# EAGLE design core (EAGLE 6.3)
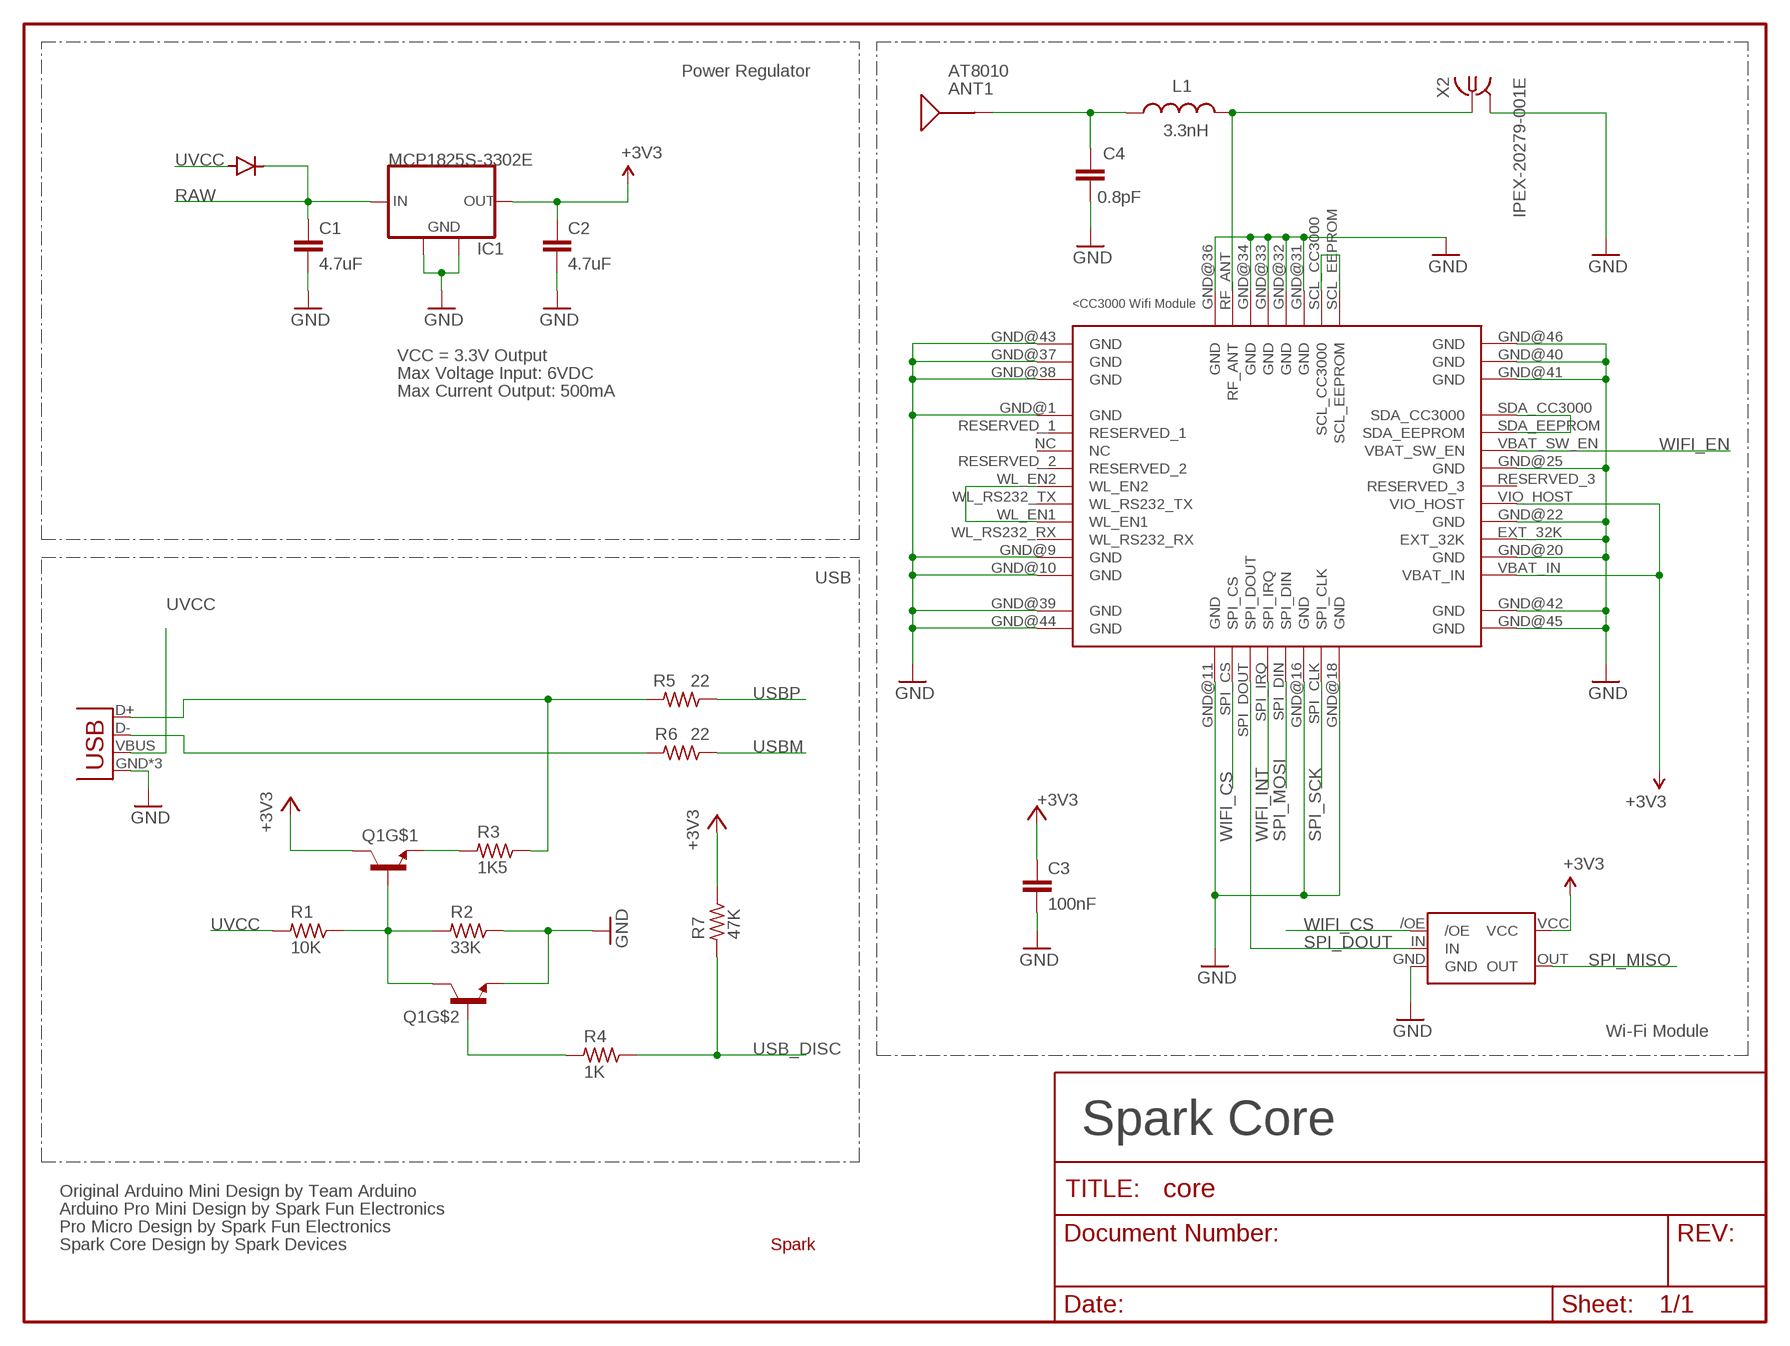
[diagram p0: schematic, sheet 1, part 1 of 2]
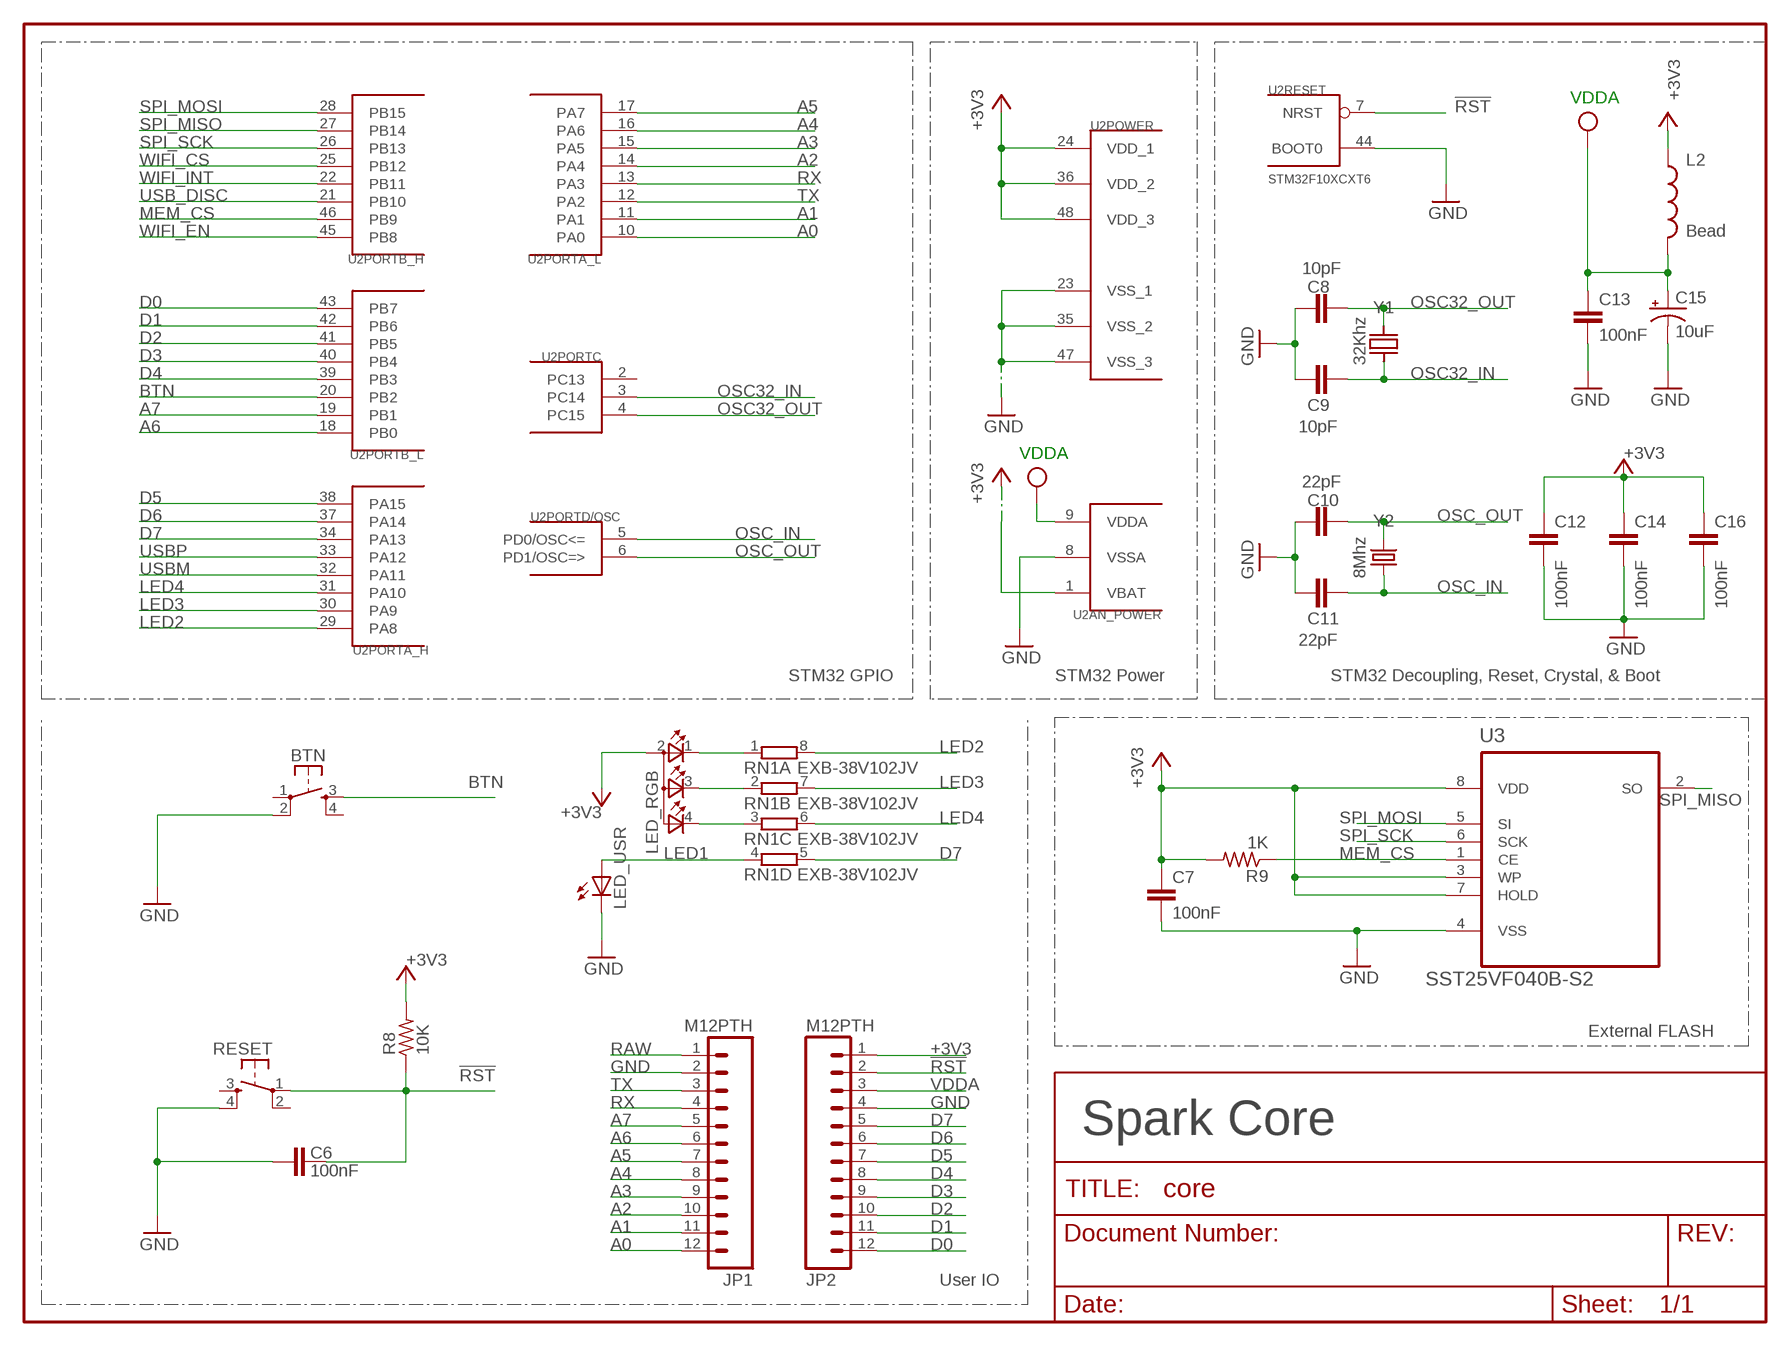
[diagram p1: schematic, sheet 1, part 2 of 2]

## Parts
ANT1  AT8010  [AT8010]
BTN  KMR211GLFS  TAC_SWITCHSMD  [TACTILE_SWITCH_SMD]
C1  4.7uF  C-EUC0603  [C0603]
C2  4.7uF  C-EUC0603  [C0603]
C3  100nF  C-EUC0603  [C0603]
C4  0.8pF  C-EUC0603  [C0603]
C6  100nF  C-EUC0603  [C0603]
C7  100nF  C-EUC0603  [C0603]
C8  10pF  C-EUC0603  [C0603]
C9  10pF  C-EUC0603  [C0603]
C10  22pF  C-EUC0603  [C0603]
C11  22pF  C-EUC0603  [C0603]
C12  100nF  C-EUC0603  [C0603]
C13  100nF  C-EUC0603  [C0603]
C14  100nF  C-EUC0603  [C0603]
C15  10uF  TANT-CAP1206  [EIA3216]
C16  100nF  C-EUC0603  [C0603]
D1  DIODE  [DIODE-DO-220AA(SMP)]
IC1  MCP1825S-3302E  MCP1825S-SOT223  [SOT223]
JP1  M12PTH  [1X12-SMALL-PADS]
JP2  M12PTH  [1X12-SMALL-PADS]
L1  3.3nH  INDUCTOR0603  [0603]
L2  Bead  INDUCTOR0603  [0603]
LED_RGB  TOPLED-3PLCC  [P-LCC-4-3]
LED_USR  LED0603  [LED-0603]
Q1  MMDT3904  [SOT363]
R1  10K  R-US_R0603  [R0603]
R2  33K  R-US_R0603  [R0603]
R3  1K5  R-US_R0603  [R0603]
R4  1K  R-US_R0603  [R0603]
R5  22  R-US_R0603  [R0603]
R6  22  R-US_R0603  [R0603]
R7  47K  R-US_R0603  [R0603]
R8  10K  R-US_R0603  [R0603]
R9  1K  R-US_R0603  [R0603]
RESET  KMR211GLFS  TAC_SWITCHSMD  [TACTILE_SWITCH_SMD]
RN1  EXB-38V102JV  4R-NEXB38V  [EXB38V]
U1  CC3000  [CC3000]
U2  STM32F10XCXT6  [TQFP48]
U3  SST25VF040B-S2  [SOIC127P790X216-8N]
U4  NL17SZ125SOT553  [SOT-553]
U$1  SPARK_LOGO2  [SPARK_LOGO2]
X1  USB-MICROB  USBUSB-MICROB-SLOT-HOLE  [USB-MICROB-SLOT-HOLE]
X2  IPEX-20279-001E  [IPEX-20279-001E]
Y1  32Khz  Q_FC135  [FC135]
Y2  8Mhz  CRYSTAL5X3  [CRYSTAL-SMD-5X3]

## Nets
!RST: C6.2 JP2.2 R8.1 RESET.1 U2.7(RESET:NRST)
+3V3: C2.1 C3.1 C7.1 C12.1 C14.1 C16.1 IC1.3(OUT) JP2.1 L2.1 LED_RGB.2(A2) Q1.3(C) R7.1 R8.2 R9.2 U1.VBAT_IN U1.VIO_HOST U2.1(AN_POWER:VBAT) U2.24(POWER:VDD_1) U2.36(POWER:VDD_2) U2.48(POWER:VDD_3) U3.3(WP) U3.7(HOLD) U3.8(VDD) U4.VCC
A0: JP1.12 U2.10(PORTA_L:PA0)
A1: JP1.11 U2.11(PORTA_L:PA1)
A2: JP1.10 U2.14(PORTA_L:PA4)
A3: JP1.9 U2.15(PORTA_L:PA5)
A4: JP1.8 U2.16(PORTA_L:PA6)
A5: JP1.7 U2.17(PORTA_L:PA7)
A6: JP1.6 U2.18(PORTB_L:PB0)
A7: JP1.5 U2.19(PORTB_L:PB1)
BTN: BTN.3 U2.20(PORTB_L:PB2)
D0: JP2.12 U2.43(PORTB_L:PB7)
D1: JP2.11 U2.42(PORTB_L:PB6)
D2: JP2.10 U2.41(PORTB_L:PB5)
D3: JP2.9 U2.40(PORTB_L:PB4)
D4: JP2.8 U2.39(PORTB_L:PB3)
D5: JP2.7 U2.38(PORTA_H:PA15)
D6: JP2.6 U2.37(PORTA_H:PA14)
D7: JP2.5 RN1.5 U2.34(PORTA_H:PA13)
GND [vcc]: BTN.2 C1.2 C2.2 C3.2 C4.2 C6.1 C7.2 C8.2 C9.2 C10.2 C11.2 C12.2 C13.2 C14.2 C15.C(-) C16.2 IC1.2(GND) IC1.4(GND) JP1.2 JP2.4 LED_USR.C Q1.1(E) R2.1 RESET.4 U1.EXT_32K U1.GND@1(GND) U1.GND@9(GND) U1.GND@10(GND) U1.GND@11(GND) U1.GND@16(GND) U1.GND@18(GND) U1.GND@20(GND) U1.GND@22(GND) U1.GND@25(GND) U1.GND@31(GND) U1.GND@32(GND) U1.GND@33(GND) U1.GND@34(GND) U1.GND@36(GND) U1.GND@37(GND) U1.GND@38(GND) U1.GND@39(GND) U1.GND@40(GND) U1.GND@41(GND) U1.GND@42(GND) U1.GND@43(GND) U1.GND@44(GND) U1.GND@45(GND) U1.GND@46(GND) U2.8(AN_POWER:VSSA) U2.23(POWER:VSS_1) U2.35(POWER:VSS_2) U2.44(RESET:BOOT0) U2.47(POWER:VSS_3) U3.4(VSS) U4.GND X1.GND X1.MT1(GND) X1.MT2(GND) X2.2@1(GND) X2.2@2(GND)
LED1: LED_USR.A RN1.4
LED2: RN1.8 U2.29(PORTA_H:PA8)
LED3: RN1.7 U2.30(PORTA_H:PA9)
LED4: RN1.6 U2.31(PORTA_H:PA10)
MEM_CS: R9.1 U2.46(PORTB_H:PB9) U3.1(CE)
N$1: R3.1 R5.2 X1.D+
N$2 [RF]: L1.2 U1.RF_ANT X2.1
N$3 [RF]: ANT1.SIG(SIGNAL) C4.1 L1.1
N$6: R6.2 X1.D-
N$7: U1.SCL_CC3000 U1.SCL_EEPROM
N$8: Q1.2(B) R4.2
N$9: U1.WL_EN1 U1.WL_EN2
N$10: LED_RGB.1(CRED) RN1.1
N$12: LED_RGB.3(CBLUE) RN1.2
N$13: Q1.5(B) Q1.6(C) R1.1 R2.2
N$14: LED_RGB.4(CGREEN) RN1.3
N$15: U1.SDA_CC3000 U1.SDA_EEPROM
N$16: Q1.4(E) R3.2
OSC32_IN: C9.1 U2.3(PORTC:PC14) Y1.X1
OSC32_OUT: C8.1 U2.4(PORTC:PC15) Y1.X2
OSC_IN: C11.1 U2.5(PORTD/OSC:PD0/OSC<=) Y2.1
OSC_OUT: C10.1 U2.6(PORTD/OSC:PD1/OSC=>) Y2.3
RAW [vcc]: C1.1 D1.CATHODE IC1.1(IN) JP1.1
RX: JP1.4 U2.13(PORTA_L:PA3)
SPI_DOUT: U1.SPI_DOUT U4.IN
SPI_MISO: U2.27(PORTB_H:PB14) U3.2(SO) U4.OUT
SPI_MOSI: U1.SPI_DIN U2.28(PORTB_H:PB15) U3.5(SI)
SPI_SCK: U1.SPI_CLK U2.26(PORTB_H:PB13) U3.6(SCK)
TX: JP1.3 U2.12(PORTA_L:PA2)
USB_DISC: R4.1 R7.2 U2.21(PORTB_H:PB10)
USBM: R6.1 U2.32(PORTA_H:PA11)
USBP: R5.1 U2.33(PORTA_H:PA12)
UVCC: D1.ANODE R1.2 X1.VBUS
VDDA: C13.1 C15.A(+) JP2.3 L2.2 U2.9(AN_POWER:VDDA) ; supply symbol labelled VCC
WIFI_CS: U1.SPI_CS U2.25(PORTB_H:PB12) U4./OE
WIFI_EN: U1.VBAT_SW_EN U2.45(PORTB_H:PB8)
WIFI_INT: U1.SPI_IRQ U2.22(PORTB_H:PB11)
Unconnected: BTN.1 BTN.4 RESET.2 RESET.3 U1.NC U1.RESERVED_1 U1.RESERVED_2 U1.RESERVED_3 U1.WL_RS232_RX U1.WL_RS232_TX U2.2(PORTC:PC13)

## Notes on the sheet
- Power Regulator
- VDDA
- VCC = 3.3V Output
- Max Voltage Input: 6VDC
- Max Current Output: 500mA
- VDDA
- USB
- STM32 GPIO | STM32 Power | STM32 Decoupling, Reset, Crystal, & Boot
- Wi-Fi Module | External FLASH
- Spark Core | Spark Core
- Original Arduino Mini Design by Team Arduino
- Arduino Pro Mini Design by Spark Fun Electronics
- Pro Micro Design by Spark Fun Electronics
- Spark Core Design by Spark Devices
- User IO

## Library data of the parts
ANT1 = Spark:AT8010: AT8010 Series Multilayer Chip Antenna
BTN RESET = Spark:TAC_SWITCH: SMD Tactiile Switch
C1-C4 C6-C14 C16 = rcl:C-EU: CAPACITOR, European symbol
C15 = Spark:TANT-CAP: Tantalum SMT
D1 = Spark:DIODE
IC1 = Spark:MCP1825S: 500 mA, Low Voltage, Low Quiescent Current LDO Regulator
JP1 JP2 = Spark:M12: Header 12 Standard 12-pin 0.1" header. Use with straight break away headers (SKU : PRT-00116), right angle break away headers (PRT-00553), swiss pins (PRT-00743), machine pins (PRT-00117), and female headers (PRT-00115).
L1 L2 = SparkFun-Passives:INDUCTOR: Inductors
LED_RGB = Spark:TOPLED-3: Cree CLVBA-FKA
LED_USR = SparkFun:LED: LEDs
Q1 = SparkFun-DiscreteSemi:MMDT3904: Dual NPN transistor
R1-R9 = rcl:R-US_: RESISTOR, American symbol
RN1 = resistor-dil:4R-N: Array Chip Resistor Source: RS Component / Phycomp; OC_FARNELL: unknown; OC_NEWARK: unknown
U1 = CC3000:CC3000
U2 = stm32:STM32F10XCXT6: ST STM32F101/103 48pin LQFP
U3 = Spark:SST25VF040B: 4 Mbit SPI Serial Flash
U4 = Spark:NL17SZ125
U$1 = Spark:SPARK_LOGO2
X1 = Spark:USB
X2 = Spark:IPEX-20279-001E: Ultra Miniature Coaxial SMT RF Receptacle
Y1 = Spark:Q
Y2 = SparkFun-FreqCtrl:CRYSTAL: Various standard crystals. Proven footprints. Spark Fun Electronics SKU : COM-00534

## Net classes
2 RF: width 0.635 mm, clearance 0.762 mm

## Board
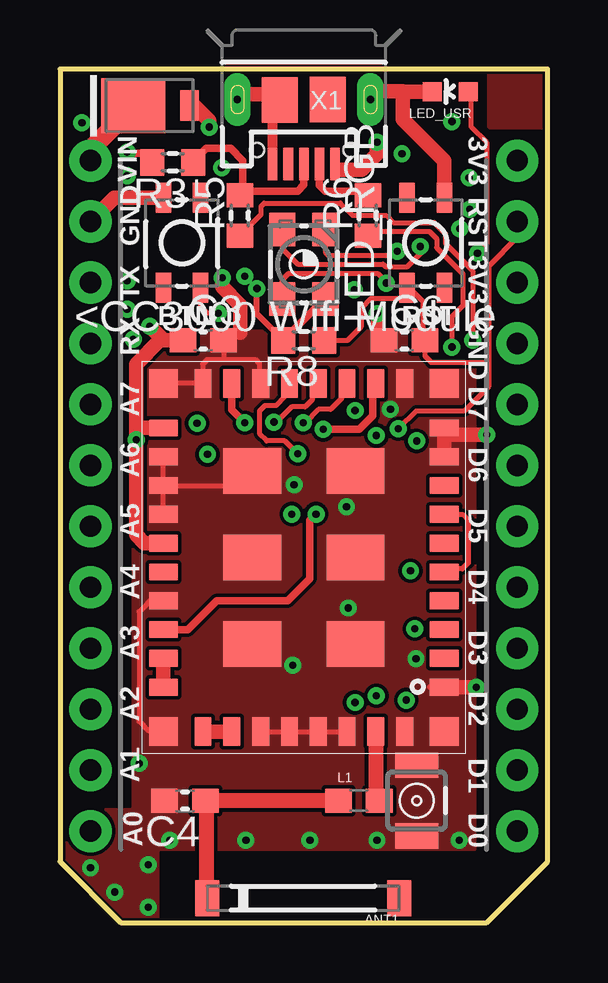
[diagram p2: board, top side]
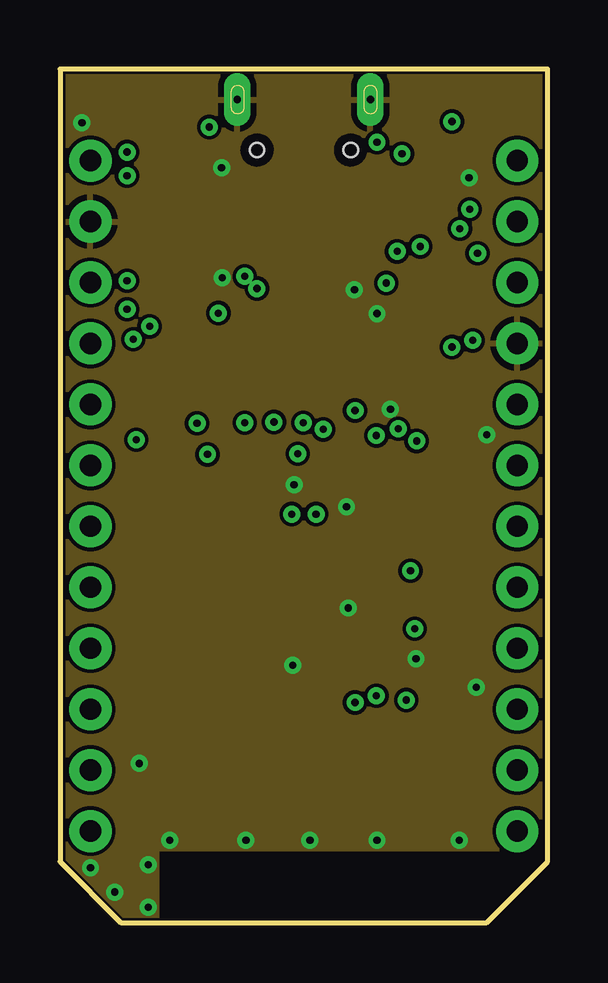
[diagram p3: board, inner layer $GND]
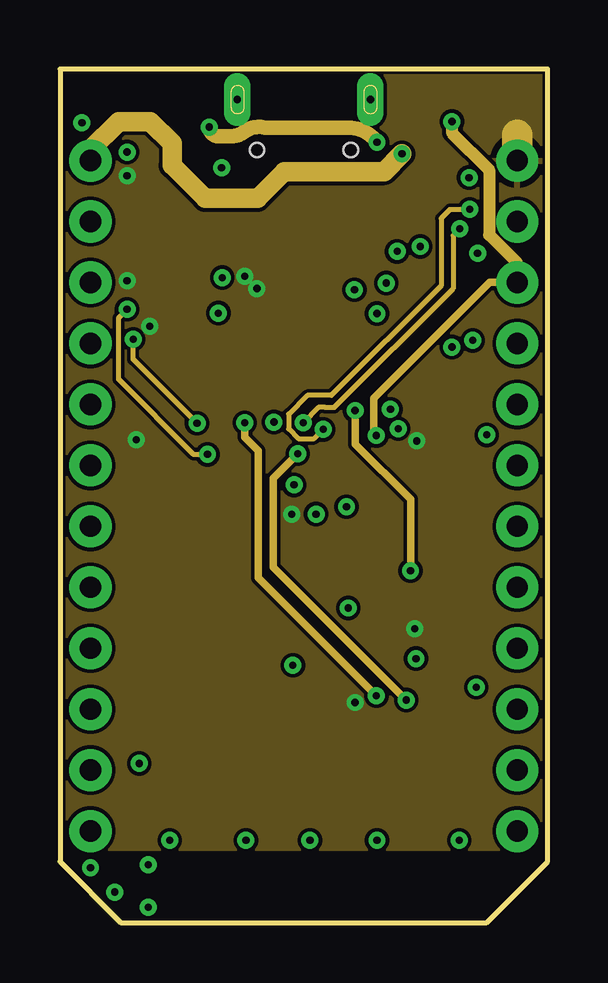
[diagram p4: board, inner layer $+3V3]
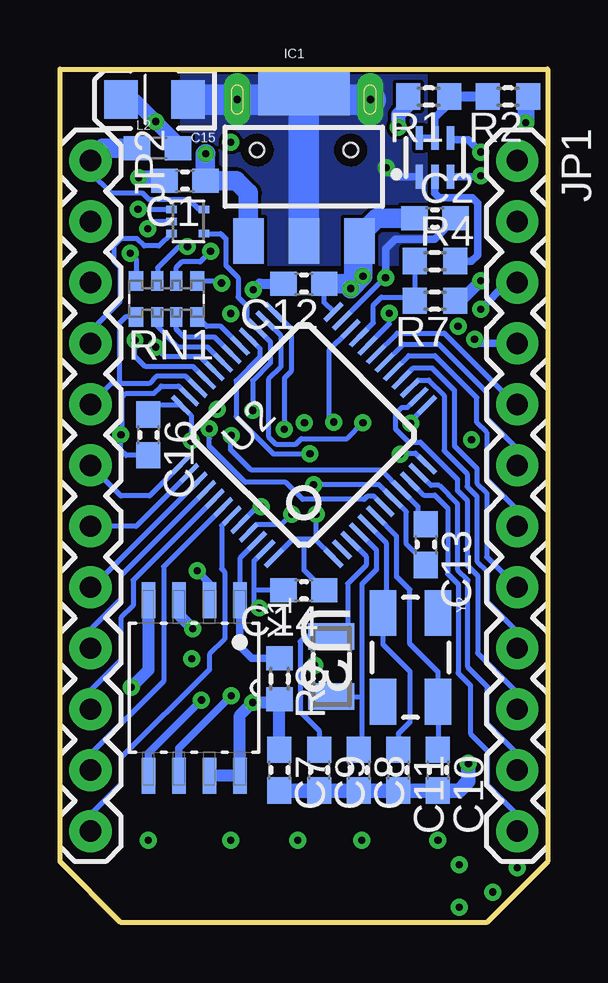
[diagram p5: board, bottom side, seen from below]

Size 20.32 x 35.56 mm. Coordinates in mm from the lower left corner, seen from the top.
Outline: 0,35.56 0,2.54 2.54,0 17.78,0 20.32,2.54 20.32,35.56 0,35.56
Copper layers (1+2*15+16): Top 0.035mm / dielectric 1.5mm / $GND 0.035mm / dielectric 0.15mm / $+3V3 0.035mm / dielectric 0.2mm / Bottom 0.035mm
Design rules "spark *": minimum track width 6mil, minimum drill 0.3mm, track to track 6mil, track to pad 6mil, pad to pad 6mil, via to via 6mil, smd to smd 6mil, copper to edge 4mil, drill to drill 6mil, minimum pad ring 12mil, minimum via ring 8mil, stop-mask expansion 4mil, vias tented up to drill 20mil, thermal gap 10mil

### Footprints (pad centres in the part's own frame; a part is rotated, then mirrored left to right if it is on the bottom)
AT8010 = smd 1 x 1.5: NC -4,0; SIG 4,0
TACTILE_SWITCH_SMD = smd 1.25 x 0.65: 1 -1.875,0.775; 2 1.875,0.775; 3 -1.875,-0.775; 4 1.875,-0.775
C0603 = smd 1.1 x 1: 1 -0.85,0; 2 0.85,0
EIA3216 = smd 1.4 x 1.6: A 1.4,0; C -1.4,0
DIODE-DO-220AA(SMP) = smd 0.762 x 1.27: ANODE 2.349,0 | smd 2.667 x 2.286: CATHODE 0,0
SOT223 = smd 1.27 x 1.905: 1 -2.311,-3.099; 2 0,-3.099; 3 2.311,-3.099 | smd 3.81 x 1.905: 4 0,3.099
1X12-SMALL-PADS = drill 0.889 pad 1.753: 1 0,0; 2 2.54,0; 3 5.08,0; 4 7.62,0; 5 10.16,0; 6 12.7,0; 7 15.24,0; 8 17.78,0; 9 20.32,0; 10 22.86,0; 11 25.4,0; 12 27.94,0
0603 = smd 1.1 x 1: 1 -0.85,0; 2 0.85,0
P-LCC-4-3 = smd 1.1 x 1.4: 1 -0.9,-1.45; 2 0.9,-1.45; 3 0.9,1.45; 4 -0.9,1.45
LED-0603 = smd 0.8 x 0.8: A 0,-0.75; C 0,0.75
SOT363 = smd 0.3 x 0.99: 1 -0.65,-0.8; 2 0,-0.8; 3 0.65,-0.8; 4 0.65,0.81; 5 0,0.81; 6 -0.65,0.81
R0603 = smd 1 x 1.1: 1 -0.85,0; 2 0.85,0
EXB38V = smd 0.6 x 0.8: 1 -1.275,-0.75; 4 1.275,-0.75; 5 1.275,0.75; 8 -1.275,0.75 | smd 0.5 x 0.8: 2 -0.4,-0.75; 3 0.4,-0.75; 6 0.4,0.75; 7 -0.4,0.75
CC3000 = smd 1.2 x 0.7: EXT_32K 5.85,-2.97; GND@1 -5.85,5.43; GND@9 -5.85,-4.17; GND@10 -5.85,-5.37; GND@20 5.85,-4.17; GND@22 5.85,-1.77; GND@25 5.85,1.83; NC -5.85,3.03; RESERVED_1 -5.85,4.23; RESERVED_2 -5.85,1.83; RESERVED_3 5.85,0.63; SDA_CC3000 5.85,5.43; SDA_EEPROM 5.85,4.23; VBAT_IN 5.85,-5.37; VBAT_SW_EN 5.85,3.03; VIO_HOST 5.85,-0.57; WL_EN1 -5.85,-1.77; WL_EN2 -5.85,0.63; WL_RS232_RX -5.85,-2.97; WL_RS232_TX -5.85,-0.57 | smd 0.7 x 1.2: GND@11 -4.2,-7.22; GND@16 1.8,-7.22; GND@18 4.2,-7.22; GND@31 1.8,7.28; GND@32 0.6,7.28; GND@33 -0.6,7.28; GND@34 -1.8,7.28; GND@36 -4.2,7.28; RF_ANT -3,7.28; SCL_CC3000 3,7.28; SCL_EEPROM 4.2,7.28; SPI_CLK 3,-7.22; SPI_CS -3,-7.22; SPI_DIN 0.6,-7.22; SPI_DOUT -1.8,-7.22; SPI_IRQ -0.6,-7.22 | smd 2.4 x 1.9: GND@37 -2.15,3.63; GND@38 -2.15,0.03; GND@39 -2.15,-3.57; GND@40 2.15,3.63; GND@41 2.15,0.03; GND@42 2.15,-3.57 | smd 1.2 x 1.2: GND@43 -5.85,7.28; GND@44 -5.85,-7.22; GND@45 5.85,-7.22; GND@46 5.85,7.28
TQFP48 = smd 0.2 x 1: 1 -2.75,-4.5; 2 -2.25,-4.5; 3 -1.75,-4.5; 4 -1.25,-4.5; 5 -0.75,-4.5; 6 -0.25,-4.5; 7 0.25,-4.5; 8 0.75,-4.5; 9 1.25,-4.5; 10 1.75,-4.5; 11 2.25,-4.5; 12 2.75,-4.5; 25 2.75,4.5; 26 2.25,4.5; 27 1.75,4.5; 28 1.25,4.5; 29 0.75,4.5; 30 0.25,4.5; 31 -0.25,4.5; 32 -0.75,4.5; 33 -1.25,4.5; 34 -1.75,4.5; 35 -2.25,4.5; 36 -2.75,4.5 | smd 1 x 0.2: 13 4.5,-2.75; 14 4.5,-2.25; 15 4.5,-1.75; 16 4.5,-1.25; 17 4.5,-0.75; 18 4.5,-0.25; 19 4.5,0.25; 20 4.5,0.75; 21 4.5,1.25; 22 4.5,1.75; 23 4.5,2.25; 24 4.5,2.75; 37 -4.5,2.75; 38 -4.5,2.25; 39 -4.5,1.75; 40 -4.5,1.25; 41 -4.5,0.75; 42 -4.5,0.25; 43 -4.5,-0.25; 44 -4.5,-0.75; 45 -4.5,-1.25; 46 -4.5,-1.75; 47 -4.5,-2.25; 48 -4.5,-2.75
SOIC127P790X216-8N = smd 1.499 x 0.559: 1 -3.658,1.905; 2 -3.658,0.635; 3 -3.658,-0.635; 4 -3.658,-1.905; 5 3.658,-1.905; 6 3.658,-0.635; 7 3.658,0.635; 8 3.658,1.905
SOT-553 = smd 0.3 x 0.45: /OE -0.5,0; GND 0.5,0; IN 0,0; OUT 0.5,1.35; VCC -0.5,1.35
USB-MICROB-SLOT-HOLE = smd 0.4 x 1.35: D+ 0,2.675; D- -0.65,2.675; GND 1.3,2.675; ID 0.65,2.675; VBUS -1.3,2.675 | drill 0.3 pad 1.1 long: MT1 -2.775,0; MT2 2.775,0 | smd 1.5 x 1.9: P$1 -1,0; P$2 1,0.01 | hole 0.6: -1.95,2.1; 1.95,2.1
IPEX-20279-001E = smd 1 x 1.05: 1 0,1.528 | smd 1.05 x 1.8: 2@1 -1.475,0; 2@2 1.475,0
FC135 = smd 1.1 x 1.9: X1 -1.25,0; X2 1.25,0
CRYSTAL-SMD-5X3 = smd 1.9 x 1.1: 1 -1.85,-1.15; 2 1.85,-1.15; 3 1.85,1.15; 4 -1.85,1.15

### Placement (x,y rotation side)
ANT1  10.13,1.02 180 top
BTN  5.08,28.32 90 top
C1  15.11,30.91 180 bottom
C2  4.7,29.34 0 bottom
C3  5.97,24.26 0 top
C4  5.21,5.08 180 top
C6  14.35,24.26 0 top
C7  11.18,6.35 270 bottom
C8  7.87,6.35 270 bottom
C9  9.53,6.35 270 bottom
C10  4.57,6.35 270 bottom
C11  6.22,6.35 270 bottom
C12  10.16,26.62 180 bottom
C13  5.08,15.75 270 bottom
C14  10.16,13.84 180 bottom
C15  16.38,34.29 180 bottom
C16  16.64,20.32 270 bottom
D1  3.05,34.04 0 top
IC1  10.16,31.5 0 bottom
JP1  1.27,31.75 270 bottom
JP2  19.05,31.75 270 bottom
L1  12.45,5.08 0 top
L2  16.26,32.26 0 bottom
LED_RGB  10.16,27.43 0 top
LED_USR  16.26,34.62 90 top
Q1  4.7,31.88 0 bottom
R1  4.95,34.42 180 bottom
R2  1.65,34.42 180 bottom
R3  4.7,31.67 180 top
R4  4.7,27.56 0 bottom
R5  7.49,29.46 90 top
R6  12.83,29.46 90 top
R7  4.7,25.91 180 bottom
R8  10.16,24.26 180 top
R9  11.18,10.16 270 bottom
RESET  15.24,28.32 90 top
RN1  15.88,25.98 180 bottom
U1  10.16,15.24 180 top
U2  10.16,20.32 45 bottom
U3  14.73,9.78 270 bottom
U4  15.67,29.21 270 bottom
U$1  17.78,33.02 0 top
X1  10.16,34.29 180 top
X2  14.86,5.08 90 top
Y1  9.02,10.67 270 bottom
Y2  5.71,11.05 270 bottom

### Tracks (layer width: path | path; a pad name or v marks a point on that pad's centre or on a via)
!RST  (via drill 0.3)
  Top 0.203: R8.1 11.99,24.26 12.55,24.82 12.55,25.6 12.95,26.01 14.46,26.01 RESET.1 14.55,26.45 15.14,25.86 15.14,24.32 C6.2 15.2,23.61 15.47,23.34 17.86,23.34 | v14.1,20.57 14.83,21.31 16.84,21.31 17.86,22.33 17.86,23.34 | JP2.2 19.05,28.55 17.86,27.36 17.86,23.34
  Bottom 0.203: 14.1,20.17 v14.1,20.57 14.1,19.84 12.6,18.34 10.92,18.34 10.21,17.63 7.64,17.63 7.49,17.78 7.27,17.78 U2.7
+3V3  (via drill 0.3)
  Top 0.254: R8.2 8.2,25.36 v8.2,26.42
  Top 0.305: R8.2 11.04,25.98 LED_RGB.2
  Top 0.61: U1.VIO_HOST 3.52,15.81 3.17,16.15 v3.17,20.12 3.17,20.62 | 3.17,20.62 3.17,23.27 4.17,24.26 4.32,24.26 | 4.32,24.26 C3.1 | U1.VBAT_IN 4.29,20.62 3.17,20.62 | v3.73,24.84 4.32,24.26
  $+3V3 1.27: JP2.1 19.05,32.82
  Bottom 0.203: U2.1 9.71,15.98 | 9.71,15.98 10.16,15.98 | 10.16,15.98 10.62,15.98 U2.48 | 10.16,15.98 10.16,14.69 C14.1 | C16.1 16.25,21.56 U2.36 14.86,21.13 v14.86,20.07 | 9.71,15.98 9.65,16.03 v9.65,17.02 | JP2.1 19.05,31.24 18.19,30.38 16.87,30.38 16.61,30.12 14.94,30.12 14.52,29.71 U4.VCC | U2.24 9.31,25.83 C12.1
  Bottom 0.305: Q1.3 2.83,31.08 arc-90 v2.79,31.11
  Bottom 0.508: U3.7 U3.8 12.83,8.64 v12.29,9.17 11.32,9.17 R9.2 C7.1 | v14.78,12.24 15.37,12.83 U3.3 | v2.79,26.75 3.63,25.91 R7.1
  Bottom 0.813: C2.1 7.11,29.34 7.85,28.6 IC1.3 7.85,27.08 v7.7,26.92 | L2.1 18.54,32.26 JP2.1 | v8.2,26.42 v7.7,26.92 | v7.7,26.92 7.7,28.83 8.08,28.45 8.08,26.62 C12.1
  pour $+3V3: 0,35.56 20.32,35.56 20.32,3.05 0,3.05
A0
  Bottom 0.203: U2.10 5.17,17.8 4.7,17.8 4.17,17.27 4.17,14.53 3.73,14.1 3.73,10.39 3.23,9.88 3.23,7.87 2.52,7.16 2.52,5.74 1.27,4.5 JP1.12
A1
  Bottom 0.203: U2.11 4.87,18.21 4.52,18.21 3.76,17.45 3.76,14.71 3.33,14.28 3.33,10.64 2.52,9.83 2.52,8.28 1.27,7.04 JP1.11
A2
  Bottom 0.203: JP1.10 1.27,9.58 2.92,11.23 2.92,14.45 3.35,14.88 3.35,17.6 3.76,18.01 3.76,18.47 5.31,20.02 5.79,20.02 6.35,20.57 6.35,21.18 6.07,21.46 5.84,21.46 U2.14
A3
  Bottom 0.203: U2.15 5.4,22.61 4.95,22.61 4.32,21.97 4.32,19.66 3.35,18.69 3.35,18.16 2.95,17.75 2.95,15.06 2.52,14.63 2.52,13.36 1.27,12.12 JP1.9
A4
  Bottom 0.203: U2.16 5.6,23.11 4.83,23.11 3.89,22.17 3.89,19.86 2.95,18.92 2.95,18.31 2.54,17.91 2.54,15.24 JP1.8
A5
  Bottom 0.203: U2.17 5.8,23.62 4.7,23.62 2.95,21.87 2.95,20.83 2.54,20.42 2.54,18.47 1.27,17.2 JP1.7
A6
  Bottom 0.203: U2.18 6.02,24.11 4.55,24.11 2.54,22.1 2.54,21.01 1.27,19.74 JP1.6
A7
  Bottom 0.203: U2.19 6.27,24.56 4.32,24.56 1.35,21.59 JP1.5
BTN  (via drill 0.3)
  Top 0.203: 5.84,26.43 BTN.3 5.87,26.43 5.87,25.65 6.13,25.39 v6.6,25.39
  Bottom 0.203: U2.20 6.6,24.94 v6.6,25.39
D0
  Bottom 0.203: JP2.12 19.05,4.5 17.78,5.77 17.78,6.86 14.1,10.54 14.1,11.18 13.46,11.81 13.46,14.61 13.59,14.73 13.59,16.54 U2.43
D1
  Bottom 0.203: U2.42 16,14.83 16,10.06 19.05,7.01 JP2.11
D2
  Bottom 0.203: U2.41 17.27,14.27 17.27,13.21 17.78,12.7 17.78,10.92 19.05,9.65 JP2.10
D3
  Bottom 0.203: U2.40 17.77,14.48 17.78,14.48 17.78,13.46 19.05,12.19 JP2.9
D4
  Bottom 0.203: U2.39 18.98,13.97 JP2.8
D5
  Bottom 0.203: U2.38 17.15,16.51 JP2.7
D6
  Bottom 0.203: U2.37 16.59,17.78 17.78,17.78 JP2.6
D7
  Bottom 0.203: 17.88,22.45 16.61,22.45 16.31,22.76 15.07,22.76 U2.34 | 17.88,22.45 18.19,22.45 JP2.5 | RN1.5 17.59,25.23 17.86,24.97 17.86,22.48 17.88,22.45
GND  (via drill 0.3)
  Top 0.203: U1.GND@43 16.01,8.12 | U1.GND@1 15.4,9.81 | U1.GND@34 U1.GND@33 U1.GND@32 U1.GND@31 8.36,8.4 | U1.GND@22 U1.EXT_32K | U1.GND@38 12.41,15.11 | U1.GND@25 4.49,13.59 3.94,13.59 3.3,12.95 3.3,8.38 3.68,8 4.27,8 U1.GND@46 | U1.EXT_32K U1.GND@20 | U1.EXT_32K 7.41,18.21 U1.GND@42 | 6.83,23.47 6.15,23.47 5.94,23.27 5.94,22.48 | 6.83,23.47 8.13,23.47 8.31,23.29 8.31,22.51 U1.GND@16 8.26,22.36 8.26,21.97 | C3.2 6.82,23.48 6.83,23.47 | U1.GND@18 5.94,22.48 | 5.94,22.48 4.33,22.48 U1.GND@45
  Top 0.406: X1.GND 8.86,34.51
  Top 0.508: v13.21,25.38 13.21,24.55 C6.1
  Top 0.61: U1.GND@1 v17.34,9.81 v17.35,9.8 | v6.76,26.87 6.76,26.49 7.52,25.73 7.52,24.57 | U1.GND@9 U1.GND@10 16.3,20.32 v17.78,20.32 | BTN.2 2.26,30.2 JP1.2 | 8.86,34.51 7.61,34.51 X1.MT2 | 14.28,34.65 13.29,34.65 X1.MT1 | RESET.4 16.02,31.74 14.28,33.48 14.28,34.65 | LED_USR.C 14.3,34.62 14.28,34.65
  $GND 0.406: X1.MT2 7.38,34.85 7.39,34.85 7.39,34.67 | X1.MT1 12.93,34.31 | 12.93,34.85 12.93,34.7
  $GND 1.016: 7.39,34.85 7.39,34.67 7.39,33.73 | 12.93,34.85 12.93,34.7 12.93,34.31 12.93,33.73
  $+3V3 0.406: 7.39,34.7 7.38,34.7 X1.MT2 | 12.93,34.7 12.94,34.7 X1.MT1
  $+3V3 0.813: 7.39,33.91 7.39,34.7 | 12.93,33.91 12.93,34.7
  Bottom 0.203: U2.35 15.37,22.35 16.1,22.35 16.41,22.05 17.58,22.05 17.73,21.89 17.73,20.37 v17.78,20.32 17.78,19.68 17.57,19.47 C16.2 | U2.47 12.24,15.05 12.24,13.84 | C13.2 5.08,14.96 5.89,15.77 5.89,17.11 U2.8 7.02,18.24 v9.75,18.24 | U4.GND 16.19,28.19 16.82,28.19 17.12,28.5 17.78,28.5 18.09,28.19 18.09,27.58 17.83,27.33 17.83,25.86 19.05,24.64 JP2.4 | U2.44 12.1,17.32 v11.94,17.32 | 12.24,13.84 12.24,13.34 v12.01,13.11 | C14.2 12.24,13.84 | U2.23 6.79,26.87 v6.76,26.87
  Bottom 0.305: 10.16,34.67 IC1.4 | Q1.1 6.36,31.08 v6.73,31.45 | C2.2 4.71,28.47 6.35,28.47 6.76,28.07 v6.76,26.87
  Bottom 0.406: v12.27,26.36 12.01,26.62 C12.2 | X1.MT2 7.37,34.29
  Bottom 0.508: U3.4 16.64,10.52 v17.35,9.8
  Bottom 0.61: C7.2 C9.2 C8.2 C11.2 C10.2 3.69,5.5 3.3,5.89 v3.3,6.63 | C1.2 16.09,31.04 v17.04,31.04
  Bottom 0.711: R2.1 0.91,34.3 v0.91,33.33
  Bottom 0.813: 10.16,34.8 IC1.4
  Bottom 1.27: IC1.2 IC1.4 | 7.37,34.29 X1.MT2 X1.MT1 C15.C
  other vias: 3.68,0.64 10.41,3.43 13.21,3.43 16.64,3.43 13.77,21.39 9.7,10.72 14.83,11 7.75,3.43 4.57,3.43 3.68,2.41 1.27,2.29 2.29,1.27
  pour $GND: 0,35.56 20.32,35.56 20.45,3.05 0.13,3.05
  pour Top (no thermals): 3.05,3.05 3.05,24.64 17.27,24.64 17.27,3.05
  pour Bottom (no thermals): 5.08,35.56 15.24,35.56 15.24,27.43 5.08,27.43
  pour Top (no thermals): 0,4.7 0,2.54 2.54,0 4.06,0 4.06,4.7
  pour $GND (no thermals): 0,4.7 0,2.54 2.54,0 4.06,0 4.06,4.7
LED1  (via drill 0.3)
  Top 0.203: v17.4,27.89 17.78,28.27 17.78,32.51 17.14,33.15 17.14,34.48 LED_USR.A
  Bottom 0.203: v17.4,27.89 17.15,27.64 RN1.4
LED2
  Bottom 0.203: U2.29 13.61,24.84 14.21,24.84 RN1.8
LED3
  Bottom 0.203: U2.30 13.85,24.36 13.87,24.38 15.14,24.38 15.47,24.72 RN1.7 15.34,25.1
LED4
  Bottom 0.203: U2.31 14.17,23.98 15.39,23.98 16.27,24.86 RN1.6
MEM_CS
  Bottom 0.203: U2.46 12.83,15.18 U3.1
  Bottom 0.305: U3.1 12.83,11.51 12.33,11.01 R9.1
N$1
  Top 0.305: X1.D+ 10.16,30.73 9.91,30.48 7.66,30.48 R5.2 7.62,30.44 7.62,31.75 7.11,32.26 6.1,32.26 5.55,31.71 R3.1
N$2
  Top 0.203: L1.2 X2.1
  Top 0.635: U1.RF_ANT 13.16,5.22 L1.2
N$3
  Top 0.635: ANT1.SIG | 6.1,5.08 6.1,1.05 ANT1.SIG | L1.1 6.1,5.08 | 6.1,5.08 C4.1
N$4
  cutout $GND: 7.52,32.19 arc-90 8.21,32.88 8.22,32.88 arc-91 8.9,32.19 arc-88 8.21,31.5 arc-92
N$6
  Top 0.305: X1.D- 10.81,30.72 11.05,30.48 12.66,30.48 R6.2
N$7
  Top 0.61: U1.SCL_CC3000 U1.SCL_EEPROM
N$8
  Bottom 0.305: Q1.2 4.7,30.38 4.52,30.2 3.15,30.2 2.92,29.97 2.92,27.81 3.17,27.56 R4.2
N$9
  Top 0.203: U1.WL_EN1 16.77,17.01 17.02,16.76 17.02,14.99 16.76,14.73 16.13,14.73 U1.WL_EN2
N$10  (via drill 0.3)
  Top 0.203: LED_RGB.1 9.26,26.79 9.53,27.05 13.23,27.05 13.59,26.7 v13.59,26.64
  Bottom 0.203: RN1.1 13.68,26.73 v13.59,26.64
N$11
  pour Top: 17.91,35.56 20.32,35.56 20.32,33.15 17.91,33.15
N$12  (via drill 0.3)
  Top 0.203: LED_RGB.3 11.06,27.93 11.18,27.81 13.89,27.81 v14.05,27.96
  Bottom 0.203: 14.07,27.94 v14.05,27.96 14.48,27.53 15.24,27.53 15.49,27.28 15.49,26.75 RN1.2
N$13
  Bottom 0.305: Q1.6 Q1.5 4.7,33.53 4.1,34.12 R1.1
  Bottom 0.406: R2.2 R1.1
N$14  (via drill 0.3)
  Top 0.203: LED_RGB.4 9.26,28.08 9.91,27.43 13.46,27.43 13.56,27.33 14.48,27.33 15.01,27.86 v15.01,28.17
  Bottom 0.203: RN1.3 16.26,26.75 16.26,27.28 15.37,28.17 v15.01,28.17
N$15
  Top 0.61: U1.SDA_EEPROM U1.SDA_CC3000
N$16  (via drill 0.3)
  Top 0.305: R3.2 3.47,32.05 2.85,32.05 v2.79,32.11
  Bottom 0.305: Q1.4 3.98,32.61 3.3,32.61 v2.79,32.11
N$17
  cutout $GND: 11.42,32.19 arc-90 12.11,32.88 12.12,32.88 arc-91 12.8,32.19 arc-88 12.11,31.5 arc-92
N$18
  cutout $+3V3: 7.52,32.19 arc-90 8.21,32.88 8.22,32.88 arc-91 8.9,32.19 arc-88 8.21,31.5 arc-92
N$19
  cutout $+3V3: 11.42,32.19 arc-90 12.11,32.88 12.12,32.88 arc-91 12.8,32.19 arc-88 12.11,31.5 arc-92
N$20
  cutout Bottom: 7.52,32.19 arc-90 8.21,32.88 8.22,32.88 arc-91 8.9,32.19 arc-88 8.21,31.5 arc-92
N$21
  cutout Bottom: 11.42,32.19 arc-90 12.11,32.88 12.12,32.88 arc-91 12.8,32.19 arc-88 12.11,31.5 arc-92
N$22
  cutout $+3V3: 6.82,34.85 arc-90 7.38,35.41 7.39,35.41 arc-90 7.95,34.85 7.95,33.76 7.95,33.73 arc-90 7.39,33.17 arc-90 6.82,33.74
  cutout $+3V3: 12.37,34.85 arc-90 12.93,35.41 12.94,35.41 arc-90 13.5,34.85 13.5,33.76 13.5,33.73 arc-90 12.94,33.17 arc-90 12.37,33.74
OSC32_IN
  Bottom 0.203: U2.3 7.57,15.25 7.57,14.88 8.33,14.12 8.33,12.27 8.43,12.17 8.77,12.17 Y1.X1 10.1,11.92 10.31,11.71 10.31,8.79 9.53,8 C9.1
OSC32_OUT
  Bottom 0.203: U2.4 7.14,15.53 7.14,14.71 7.75,14.1 7.75,9.42 | 7.75,9.42 7.75,7.33 C8.1 | Y1.X2 7.75,9.42
OSC_IN
  Bottom 0.203: U2.5 6.73,15.83 6.73,13.03 Y2.1 6.87,11.59 5.74,10.46 5.74,8.36 6.22,7.87 C11.1
OSC_OUT
  Bottom 0.203: U2.6 6.3,16.11 6.3,14.43 5.74,13.87 5.74,11.61 4.57,10.43 Y2.3 | 4.57,9.21 Y2.3 | Y2.3 C10.1
RAW  (via drill 0.3)
  Top 0.813: D1.CATHODE 3.05,33.98 1.27,32.21 JP1.1
  $+3V3 0.813: v14.25,32.03 13.51,31.29 9.35,31.29 8.23,30.18 6.04,30.18 4.67,31.55 4.67,32.46 3.76,33.38 2.44,33.38 1.27,32.21 JP1.1
  Bottom 0.813: IC1.1 12.47,30.4 12.98,30.91 C1.1 14.26,32.02 v14.25,32.03
RX  (via drill 0.3)
  $+3V3 0.203: v5.71,20.8 3.05,23.47 v3.05,24.31
  Bottom 0.203: U2.13 5.71,20.88 v5.71,20.8
  Bottom 0.305: JP1.4 2.87,24.13 v3.05,24.31
SPI_DOUT  (via drill 0.3)
  Top 0.203: U1.SPI_DOUT 11.73,22.23 11.73,21.84 11.28,21.39 10.77,21.39 10.21,20.83 v10.13,20.83
  $+3V3 0.203: v16.66,28.91 16.38,28.63 16.38,26.42 11.43,21.46 11.05,21.46 10.77,21.46 v10.13,20.83
  Bottom 0.203: U4.IN 16.36,29.21 v16.66,28.91
SPI_MISO  (via drill 0.3)
  $+3V3 0.305: v12.29,21.34 12.29,19.94 14.61,17.63 v14.61,14.66
  Bottom 0.203: v12.29,21.34 12.29,22.58 11.56,23.32 11.56,24.19 U2.27 12.55,25.18 12.55,25.7 12.9,26.06 12.9,26.87 13.41,27.38 13.41,28.5 13.62,28.71 U4.OUT
  Bottom 0.305: U3.2 14.1,14.15 v14.61,14.66 | v12.29,21.34 12.32,21.34
SPI_MOSI  (via drill 0.3)
  Top 0.203: 9.37,22.27 9.37,21.92 8.99,21.54 8.53,21.54 8.31,21.31 8.31,20.37 8.61,20.07 9.37,20.07 v9.91,19.53
  Top 0.305: U1.SPI_DIN 9.37,22.27
  $+3V3 0.305: v14.43,9.27 8.89,14.81 8.89,18.52 v9.91,19.53
  Bottom 0.203: U2.28 11.99,23.92 11.99,23.57 12.98,22.58 12.98,21.08 11.43,19.53 v9.91,19.53
  Bottom 0.305: U3.5 16.64,7.06 v14.43,9.27
SPI_SCK  (via drill 0.3)
  Top 0.305: U1.SPI_CLK 7.16,21.36 v7.7,20.83
  $+3V3 0.305: v13.18,9.45 8.26,14.38 8.26,19.66 7.7,20.22 v7.7,20.83
  Bottom 0.203: U2.26 11.12,24.47 11.12,23.14 11.63,22.63 11.63,20.24 11.33,19.94 10.49,19.94 10.26,20.17 8.36,20.17 v7.7,20.83
  Bottom 0.305: U3.6 15.37,7.26 v13.18,9.45
TX  (via drill 0.3)
  $+3V3 0.203: v2.79,25.55 2.44,25.2 2.44,22.63 5.56,19.51 v6.15,19.51
  Bottom 0.203: U2.12 5.51,19.56 6.1,19.56 v6.15,19.51
  Bottom 0.305: v2.79,25.55 1.68,26.67 JP1.3
USB_DISC
  Bottom 0.203: U2.21 7.26,24.98 7.26,25.73 6.93,26.06 5.7,26.06 R7.2 R4.1
USBM  (via drill 0.3)
  Top 0.203: 12.94,28.73 R6.1 arc-90 13.04,28.83 13.07,28.8 15.39,28.8 15.7,28.5 15.7,28.12 16.79,27.03 16.79,25.7 16.33,25.25 v16.33,23.98
  Bottom 0.203: U2.32 14.47,23.57 15.93,23.57 v16.33,23.98
USBP  (via drill 0.3)
  Top 0.203: 7.42,28.54 R5.1 8.38,29.5 8.38,29.84 8.51,29.97 11.68,29.97 12.19,29.46 13.59,29.46 13.89,29.16 15.6,29.16 16.05,28.7 16.05,28.3 17.2,27.15 v17.2,24.26
  Bottom 0.203: U2.33 14.77,23.16 16.76,23.16 17.2,23.6 v17.2,24.26
UVCC  (via drill 0.3)
  Top 0.305: X1.VBUS 11.44,31.61 arc-90 11.43,31.62 11.68,31.37
  Top 0.61: D1.ANODE 5.59,34.04 6.22,33.4 v6.22,33.15 | 11.68,31.37 12.57,31.37 13.21,32 v13.21,32.51
  $+3V3 0.61: v6.22,33.15 arc90 6.6,32.77 7.14,32.77 arc37 7.67,32.94 arc-50 8.53,33.12 12.01,33.12 arc-54 v13.21,32.51
  Bottom 0.61: R1.2 5.8,34.08 6.22,33.66 v6.22,33.15
VDDA  (via drill 0.3)
  $+3V3 0.305: v13.18,20.3 13.08,20.4 13.08,21.84 17.91,26.67 JP2.3
  $+3V3 0.508: v16.33,33.38 16.33,32.92 17.88,31.37 17.88,28.65 19.05,27.48 JP2.3
  Bottom 0.203: C13.1 5.41,16.93 5.41,17.34 U2.9 6.92,18.85 12.34,18.85 13.21,19.71 13.21,20.27 v13.18,20.3
  Bottom 0.61: L2.2 15.41,32.45 v16.33,33.38 17.2,34.24 17.73,34.24
  Bottom 0.762: 17.8,34.27 C15.A
  Bottom 0.813: 17.73,34.24 C15.A
WIFI_CS  (via drill 0.3)
  Top 0.203: U1.SPI_CS 12.91,22.7
  Top 0.305: v10.97,20.55 12.47,20.55 13.03,21.11 13.03,22.33 U1.SPI_CS
  $+3V3 0.203: v10.97,20.55 10.59,20.17 9.93,20.17 9.53,20.57 9.53,21.18 10.31,21.97 11.3,21.97 15.88,26.54 15.88,29.34 16.26,29.72 v17.07,29.72
  Bottom 0.203: U2.25 10.69,24.74 10.69,22.96 10.97,22.68 v10.97,20.55 | U4./OE v17.06,29.71 v17.07,29.72
WIFI_EN  (via drill 0.3)
  Top 0.203: 4.33,12.19 U1.VBAT_SW_EN
  Top 0.305: U1.VBAT_SW_EN 5.33,12.21 6.53,13.41 9.5,13.41 10.41,14.33 10.41,16.76 v10.67,17.02
  Bottom 0.203: U2.45 12.13,16.59 11.1,16.59 v10.67,17.02
WIFI_INT  (via drill 0.3)
  Top 0.203: U1.SPI_IRQ 10.76,22.14 10.52,21.89 10.52,21.79 10.21,21.49 9.65,21.49 9.02,20.85 v8.91,20.85
  Bottom 0.203: U2.22 8.72,24.23 8.74,24.23 9.09,23.88 9.09,21.03 v8.91,20.85

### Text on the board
tPlace: 3V3 | VIN | RST | GND | 3V3 | TX | BTN | RST | GND | RX | D7 | A7 | D6 | A6 | D5 | A5 | D4 | A4 | D3 | A3 | D2 | A2 | D1 | A1 | D0 | A0

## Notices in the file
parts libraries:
SparkFun-Passives: Licensing: CC v3.0 Share-Alike You are welcome to use this library for commercial purposes.
